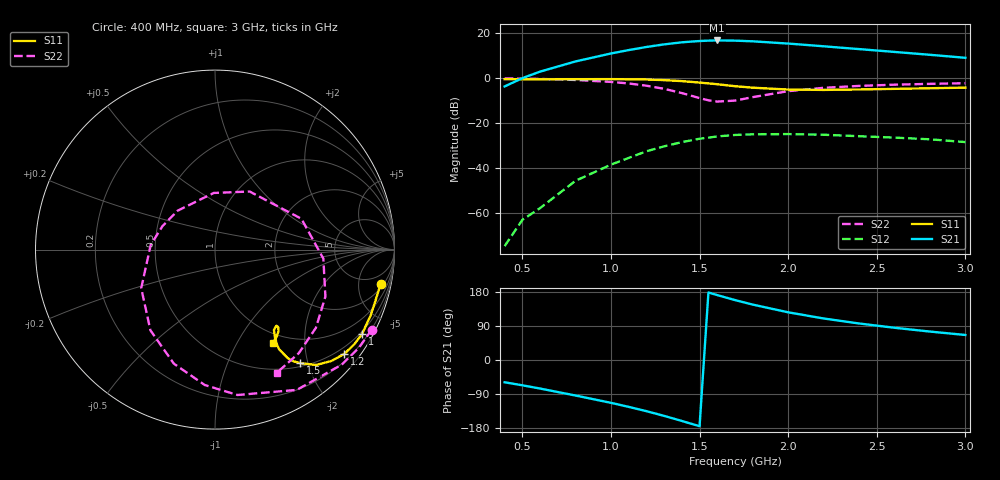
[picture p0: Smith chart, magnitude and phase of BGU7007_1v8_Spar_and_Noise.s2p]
! BGU7007, Vcc=1.80 V, Icc=4.652 mA
# MHz S MA R 50
!  Freq-MHz  S11-mag  S11-arg  S21-mag  S21-arg  S12-mag  S12-arg  S22-mag  S22-arg
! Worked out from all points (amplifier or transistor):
!   20 points, 400 MHz to 3 GHz, reference 50 ohm
!   highest |S21| = 16.6 dB at 1.6 GHz (marker M1)
!   |S21| within 3 dB of that: 1.192 GHz to 2.266 GHz (1.074 GHz wide, 62.1 % of centre)
!   unconditionally stable (mu >= 1): start of sweep to 1.121 GHz; 1.949 GHz to end of sweep
!   at 800 MHz: K = 1.47, MAG = 22.4 dB, |S12| = -45.6 dB
!   at 1.55 GHz: K = 0.93, MSG = 21.5 dB, |S12| = -26.4 dB
!   at 3 GHz: K = 1.54, MAG = 14.3 dB, |S12| = -28.4 dB
!   S11 on the Smith chart (normalised r, x): 400 MHz: 2.60, -8.97; 1 GHz: 0.42, -3.70; 1.2 GHz: 0.34, -2.80; 1.5 GHz: 0.55, -1.88; 3 GHz: 0.85, -1.42
400  0.9428 -11.8  0.6501 -58.8  0.000188 -75.1  0.9806 -27.0
500  0.9393 -14.4  0.9922 -66.8  0.0007188 -83.5  0.9705 -34.4
600  0.9383 -16.9  1.385 -75.3  0.001311 -101.7  0.9536 -42.2
800  0.9415 -22.8  2.329 -93.7  0.005277 -126.2  0.9049 -59.7
1000  0.9447 -29.9  3.497 -113.0  0.01203 -146.2  0.8197 -81.2
1100  0.9383 -34.1  4.158 -123.6  0.01695 -156.1  0.7566 -94.3
1200  0.926 -38.8  4.871 -135.0  0.02379 -168.2  0.6757 -109.8
1300  0.8977 -43.7  5.557 -147.4  0.03061 179.2  0.5761 -128.7
1400  0.8546 -48.8  6.179 -160.8  0.03793 166.1  0.4636 -152.4
1500  0.792 -53.0  6.607 -174.8  0.04515 152.2  0.3591 175.8
1550  0.7606 -54.9  6.732 178.2  0.04764 144.7  0.3206 155.9
1600  0.7283 -56.2  6.793 171.3  0.05079 137.8  0.3005 133.9
1700  0.6589 -57.2  6.731 158.1  0.05468 125.1  0.3156 91.3
1800  0.6109 -56.5  6.503 146.2  0.05656 113.3  0.3768 59.2
2000  0.5546 -53.7  5.795 125.8  0.05722 94.0  0.5113 19.6
2200  0.5449 -51.1  5.042 109.5  0.05532 79.3  0.6057 -4.7
2400  0.5573 -50.8  4.372 96.4  0.05132 68.4  0.6684 -23.0
2600  0.5749 -52.0  3.784 85.0  0.04779 58.2  0.7113 -37.8
2800  0.5934 -54.4  3.268 75.0  0.04387 51.3  0.7423 -51.0
3000  0.6119 -58.3  2.805 66.0  0.03805 45.5  0.7674 -63.3
